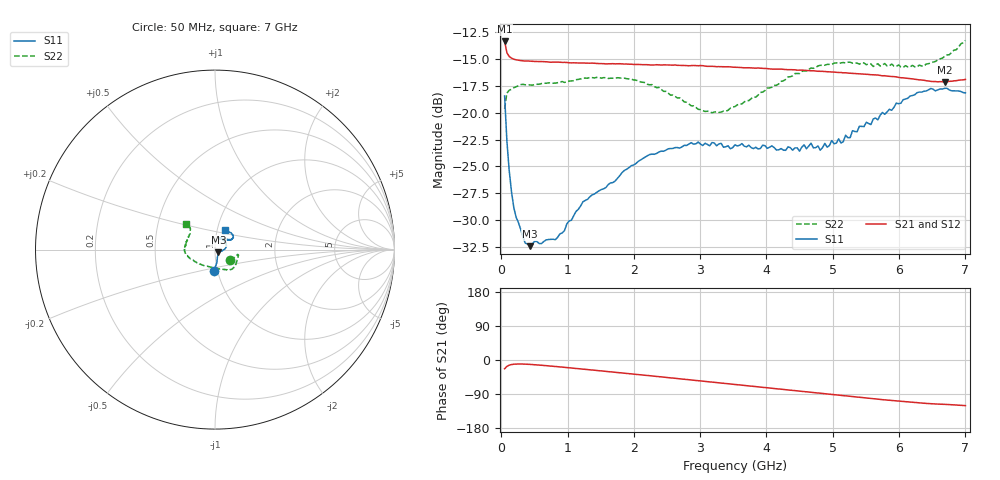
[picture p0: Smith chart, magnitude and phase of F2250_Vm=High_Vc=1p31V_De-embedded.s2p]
! Integrated Device Technology
! Corporate Headquarters
! 6024 Silver Creek Valley Road
! San Jose, CA 95138  USA
! Phone:  1-408-284-8200
! Toll Free:  1-800-223-1366
! Webpage:  http://www.idt.com/
! Timing and RF Division
! 515 Groton Road, Suite 102
! Westford, MA 01886-6024
! Device:  F2250
! Description: Voltage Variable RF Attenuator
! Frequency:  50.0 -  6000.00 MHz
! Package:  3x3 mm Thin QFN Plastic Package: 16 pin
! Ports:  2 RF, 3 DC
!  Pin  1  = GND
!  Pin  2  = NC
!  Pin  3  = RF1  = Port 1
!  Pin  4  = NC
!  Pin  5  = GND
!  Pin  6  = GND
!  Pin  7  = GND
!  Pin  8  = GND
!  Pin  9  = NC
!  Pin 10  = RF2  = Port 2
!  Pin 11  = NC
!  Pin 12  = GND
!  Pin 13  = GND
!  Pin 14  = VCNTRL
!  Pin 15  = VDD
!  Pin 16  = VMODE
! Vcntrl:  1.310 Volts
! Vmode:  +3.300 Volts
! Vdd:  +3.30  Volts
! Current:  1.332 mA
! Data:  The device was measured on a the F2250 evaluation board which has
!  individual transmission lines to the RF pins.  Data was collected
!  using a calibrated network analyzer.  The evaluation board was
!  de-embedded using a TRL calibration technique.
!  The reference plane is the edge of the package pin.
! Misc:  SN 10
!  Action Tracker AT0258
! Date Measured:  2014-11-26
! Date:  2015-10-15  MJV
! Note:
!  Integrated Device Technology supplies this data as a sample of measured
!  data at the package pin for this product.  Your particular data for this
!  product may vary.
!  Data was taken at 25 degrees C.
!  Integrated Device Technology reserves the right to change this data at anytime.
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# GHz S dB R 50
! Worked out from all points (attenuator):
!   201 points, 50 MHz to 7 GHz, reference 50 ohm
!   highest |S21| = -13.41 dB at 50 MHz (marker M1); lowest = -17.2 dB at 6.687 GHz (marker M2)
!   lowest |S11| = -32.4 dB at 432.2 MHz (marker M3), VSWR 1.05, Z = 51.9 - j1.5 ohm
!   |S11| at or under -10 dB: start of sweep to end of sweep
!   |S22| runs from -20.0 to -13.3 dB; largest |S21 - S12| = 0.00084
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0.05  -18.47 -93.3  -13.41 -23.2  -13.41 -23.2  -19.67 -35.6
0.08475  -22.66 -82.0  -14.46 -16.8  -14.45 -16.8  -18.19 -18.1
0.1195  -25.39 -76.7  -14.81 -13.6  -14.80 -13.6  -17.93 -13.4
0.189  -28.82 -64.9  -15.06 -11.1  -15.07 -11.1  -17.70 -12.0
0.36275  -32.10 -40.5  -15.23 -10.9  -15.21 -10.9  -17.43 -13.7
0.43225  -32.38 -36.9  -15.24 -11.6  -15.23 -11.6  -17.44 -15.0
0.8145  -31.78 -17.4  -15.33 -17.1  -15.32 -17.1  -17.27 -26.6
1.2315  -28.27 -12.2  -15.41 -24.0  -15.38 -24.1  -16.81 -37.3
1.857  -25.36 2.7  -15.51 -34.8  -15.52 -34.8  -16.82 -49.3
2.37825  -23.65 16.3  -15.58 -44.0  -15.62 -44.0  -17.67 -60.5
3.07325  -22.85 38.5  -15.70 -56.5  -15.70 -56.5  -19.90 -91.7
3.525  -22.99 53.8  -15.81 -64.6  -15.82 -64.7  -19.44 -122.1
4.7065  -23.27 64.2  -16.13 -86.0  -16.14 -86.0  -15.90 -168.5
4.81075  -23.49 60.5  -16.18 -87.9  -16.18 -87.9  -15.62 -170.5
5.08875  -22.44 51.4  -16.29 -92.9  -16.27 -93.0  -15.47 -176.9
5.1235  -22.83 51.6  -16.29 -93.6  -16.29 -93.6  -15.40 -177.9
5.193  -22.10 46.9  -16.32 -94.8  -16.32 -94.8  -15.41 -179.0
5.2625  -22.32 43.3  -16.36 -96.0  -16.36 -96.0  -15.34 -180.0
5.85325  -19.70 32.8  -16.65 -106.3  -16.64 -106.4  -15.66 164.8
6.3745  -18.03 36.2  -17.01 -114.3  -17.03 -114.3  -15.70 147.7
6.68725  -17.76 45.0  -17.16 -117.1  -17.15 -117.2  -14.79 139.1
7  -18.18 63.4  -16.93 -120.4  -16.92 -120.6  -13.32 138.2
